(* Logix 5000 Program export IO_Mapping; software revision 30.00; part 2 of 3 *)
(* tags used below, declared in another part *)
   Out_VMAC : DINT[8];
   MajFunc : DINT;
   HashBuffer_H : DINT;
   HashBuffer_G : DINT;
   HashBuffer_F : DINT;
   HashBuffer_E : DINT;
   HashBuffer_D : DINT;
   HashBuffer_C : DINT;
   HashBuffer_B : DINT;
   HashBuffer_A : DINT;
   W : DINT[64];   // MESSAGE SCHEDULE
   tmp : DINT[20];
   T2 : DINT;
   T1 : DINT;
   t : INT;
   M : INT;   // MESSAGE INCREMENTS
   SigmaE : DINT;
   SigmaA : DINT;
   i : INT;
   HashBufferInput_H : DINT;
   HashBufferInput_G : DINT;
   HashBufferInput_F : DINT;
   HashBufferInput_E : DINT;
   HashBufferInput_D : DINT;
   HashBufferInput_C : DINT;
   HashBufferInput_B : DINT;
   HashBufferInput_A : DINT;
   K : DINT[64];
   TOTAL_MSG_LENGTH_MINUS_16 : DINT;
   ROUNDS : DINT;
   n : INT;
(* VMAC, continued *)

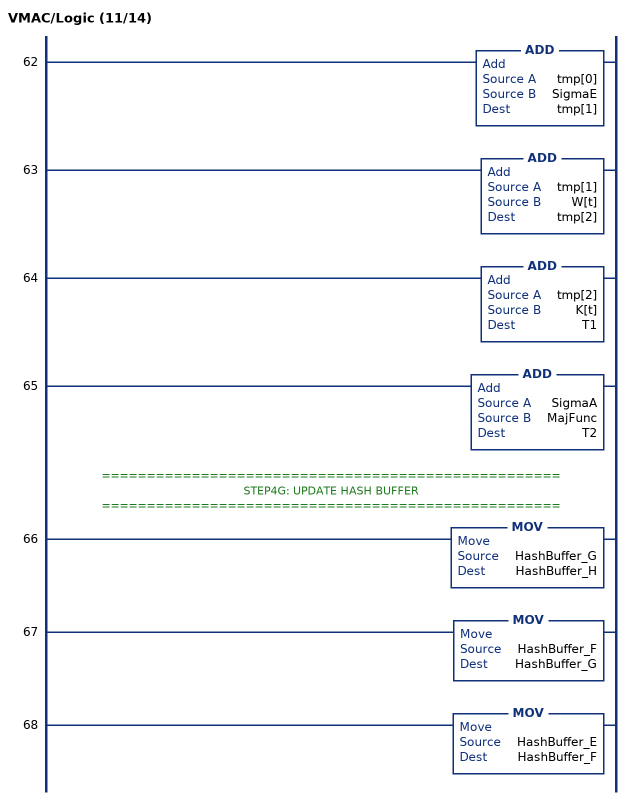
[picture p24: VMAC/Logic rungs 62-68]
   62: ADD(tmp[0],SigmaE,tmp[1]);
   63: ADD(tmp[1],W[t],tmp[2]);
   64: ADD(tmp[2],K[t],T1);
   65: ADD(SigmaA,MajFunc,T2);
   // ===================================================
   // STEP4G: UPDATE HASH BUFFER
   // ===================================================
   66: MOV(HashBuffer_G,HashBuffer_H);
   67: MOV(HashBuffer_F,HashBuffer_G);
   68: MOV(HashBuffer_E,HashBuffer_F);
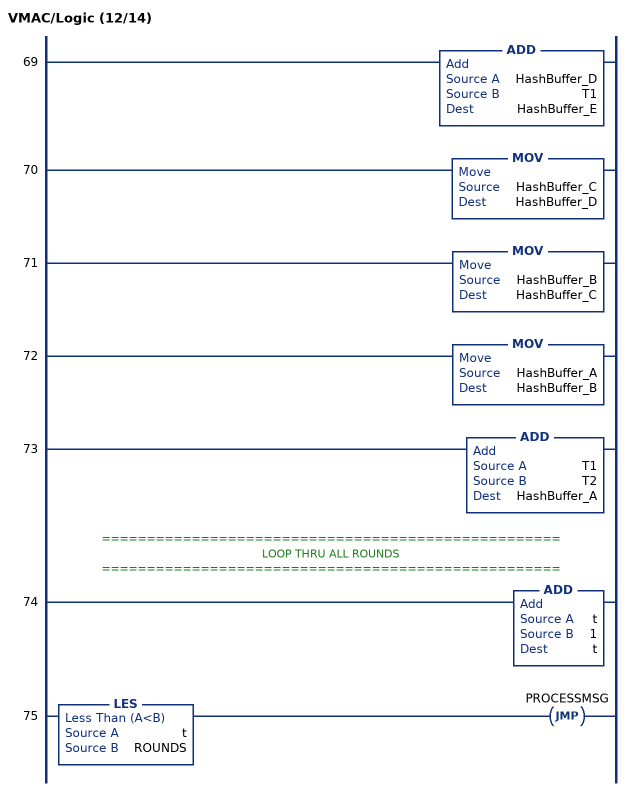
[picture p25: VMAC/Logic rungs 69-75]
   69: ADD(HashBuffer_D,T1,HashBuffer_E);
   70: MOV(HashBuffer_C,HashBuffer_D);
   71: MOV(HashBuffer_B,HashBuffer_C);
   72: MOV(HashBuffer_A,HashBuffer_B);
   73: ADD(T1,T2,HashBuffer_A);
   // ===================================================
   // LOOP THRU ALL ROUNDS
   // ===================================================
   74: ADD(t,1,t);
   75: LES(t,ROUNDS)JMP(PROCESSMSG);
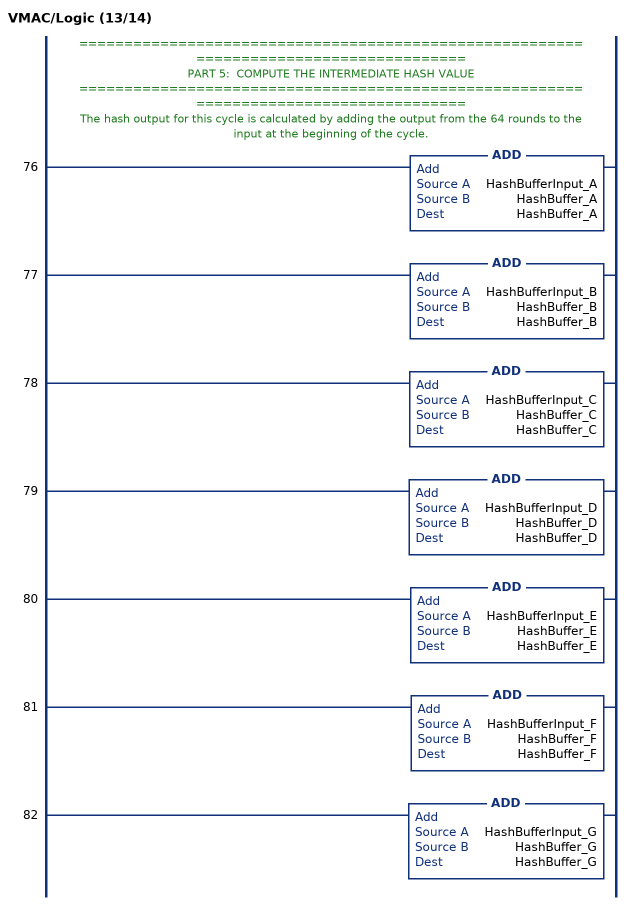
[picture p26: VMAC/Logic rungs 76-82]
   // ======================================================================================
   // PART 5:  COMPUTE THE INTERMEDIATE HASH VALUE
   // ======================================================================================
   // The hash output for this cycle is calculated by adding the output from the 64 rounds to the input at the beginning of the cycle.
   76: ADD(HashBufferInput_A,HashBuffer_A,HashBuffer_A);
   77: ADD(HashBufferInput_B,HashBuffer_B,HashBuffer_B);
   78: ADD(HashBufferInput_C,HashBuffer_C,HashBuffer_C);
   79: ADD(HashBufferInput_D,HashBuffer_D,HashBuffer_D);
   80: ADD(HashBufferInput_E,HashBuffer_E,HashBuffer_E);
   81: ADD(HashBufferInput_F,HashBuffer_F,HashBuffer_F);
   82: ADD(HashBufferInput_G,HashBuffer_G,HashBuffer_G);
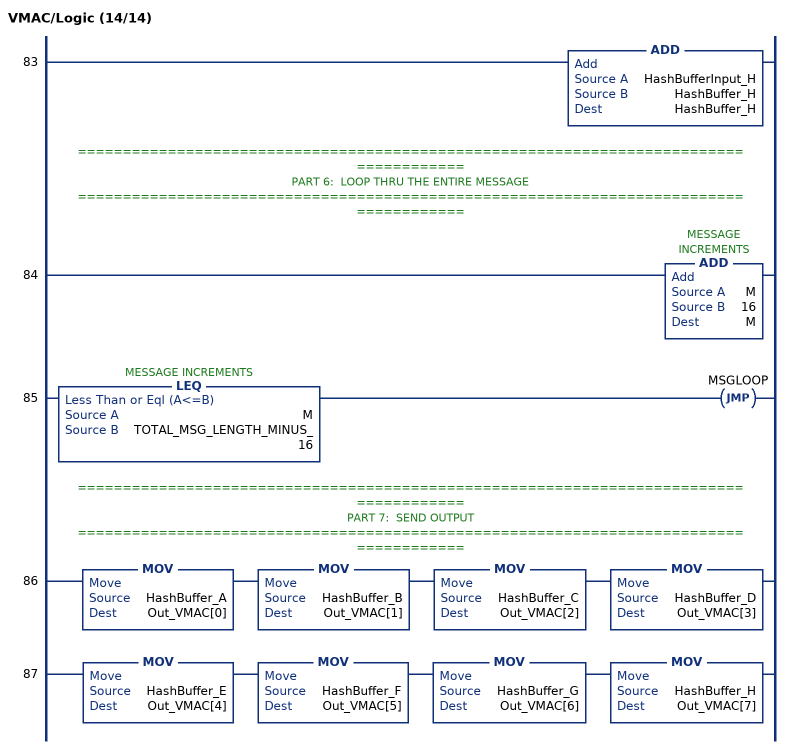
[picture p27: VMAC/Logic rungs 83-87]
   83: ADD(HashBufferInput_H,HashBuffer_H,HashBuffer_H);
   // ======================================================================================
   // PART 6:  LOOP THRU THE ENTIRE MESSAGE
   // ======================================================================================
   84: ADD(M,16,M);
   85: LEQ(M,TOTAL_MSG_LENGTH_MINUS_16)JMP(MSGLOOP);
   // ======================================================================================
   // PART 7:  SEND OUTPUT
   // ======================================================================================
   86: MOV(HashBuffer_A,Out_VMAC[0])MOV(HashBuffer_B,Out_VMAC[1])MOV(HashBuffer_C,Out_VMAC[2])MOV(HashBuffer_D,Out_VMAC[3]);
   87: MOV(HashBuffer_E,Out_VMAC[4])MOV(HashBuffer_F,Out_VMAC[5])MOV(HashBuffer_G,Out_VMAC[6])MOV(HashBuffer_H,Out_VMAC[7]);
END_ROUTINE
END_ADD_ON_INSTRUCTION

ADD_ON_INSTRUCTION L_EQU   (* revision 1.0 01 Release, vendor Rockwell Automation, ExecuteEnableInFalse *)
// Equal (64-bit)
// Revision note:
// Deleted unused Local Tag
// Help:
// This instruction compares two LINT (64-bit signed integer) variables.
// If Inp_A is equal to Inp_B, EnableOut and Out are set to true (1).
// Otherwise EnableOut and Out are cleared to false (0).
VAR_IN_OUT
   Inp_A : LINT; {required}   // Input A
   Inp_B : LINT; {required}   // Input B
END_VAR
VAR_OUTPUT
   Out : BOOL; {access Read Only, visible}   // TRUE if Inp_A is greater than or equal to Inp_B
END_VAR
VAR
   Wrk_Inp_B : DINT[2];   // 32-bit portions of Input B
   Wrk_Inp_A : DINT[2];   // 32-bit portions of Input A
END_VAR

ROUTINE EnableInFalse   (* ladder *)
// If rung is false, clear output "Out"
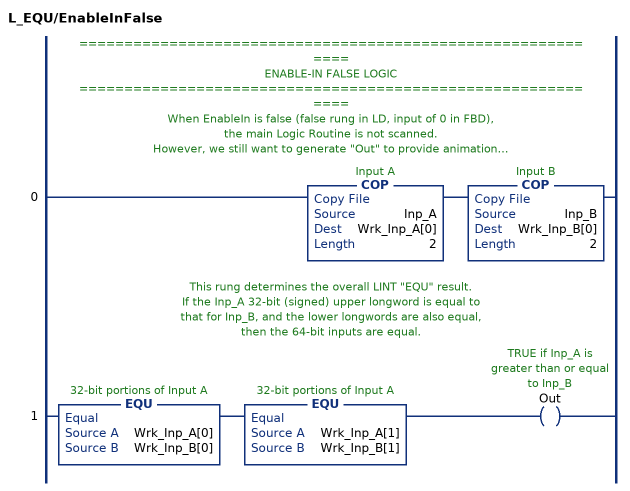
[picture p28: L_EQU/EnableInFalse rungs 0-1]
   // ============================================================
   // ENABLE-IN FALSE LOGIC
   // ============================================================
   // When EnableIn is false (false rung in LD, input of 0 in FBD),
   // the main Logic Routine is not scanned.
   // However, we still want to generate "Out" to provide animation!
   // ===================================================
   // CONVERT LINTs TO DINTs
   // ===================================================
   // These COPies take the input LINTs and break them into a
   // pair of DINTs each.  If the corresponding DINTs (high-order and high-order,
   // and low-order and low-order) are equal, then the input LINTs are equal.
   0: COP(Inp_A,Wrk_Inp_A[0],2)COP(Inp_B,Wrk_Inp_B[0],2);
   // This rung determines the overall LINT "EQU" result.
   // If the Inp_A 32-bit (signed) upper longword is equal to
   // that for Inp_B, and the lower longwords are also equal,
   // then the 64-bit inputs are equal.
   1: EQU(Wrk_Inp_A[0],Wrk_Inp_B[0])EQU(Wrk_Inp_A[1],Wrk_Inp_B[1])OTE(Out);
END_ROUTINE

ROUTINE Logic   (* ladder *)
// Compare inputs and output TRUE if they are equal
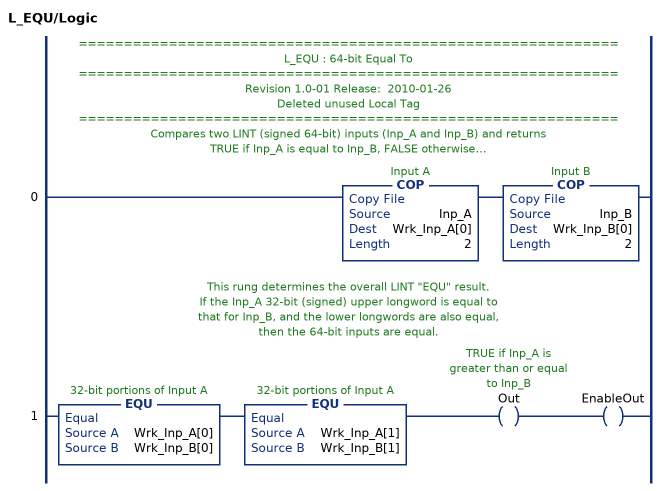
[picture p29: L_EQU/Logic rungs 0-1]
   // ============================================================
   // L_EQU : 64-bit Equal To
   // ============================================================
   // Revision 1.0-01 Release:  2010-01-26
   // Deleted unused Local Tag
   // ============================================================
   // Compares two LINT (signed 64-bit) inputs (Inp_A and Inp_B) and returns
   // TRUE if Inp_A is equal to Inp_B, FALSE otherwise.
   // This instruction breaks each LINT inputs into two DINTs
   // (32 bit signed each) to do the comparison.
   // ===================================================
   // CONVERT LINTs TO DINTs
   // ===================================================
   // These COPies take the input LINTs and break them into a
   // pair of DINTs each.  If the corresponding DINTs (high-order and high-order,
   // and low-order and low-order) are equal, then the input LINTs are equal.
   0: COP(Inp_A,Wrk_Inp_A[0],2)COP(Inp_B,Wrk_Inp_B[0],2);
   // This rung determines the overall LINT "EQU" result.
   // If the Inp_A 32-bit (signed) upper longword is equal to
   // that for Inp_B, and the lower longwords are also equal,
   // then the 64-bit inputs are equal.
   1: EQU(Wrk_Inp_A[0],Wrk_Inp_B[0])EQU(Wrk_Inp_A[1],Wrk_Inp_B[1])OTE(Out)OTE(EnableOut);
END_ROUTINE
END_ADD_ON_INSTRUCTION

ADD_ON_INSTRUCTION L_LES   (* revision 1.1 20170624, vendor Ken Fischer, NSWCPD, C516, ExecuteEnableInFalse *)
// Less Than (64-bit)
// Revision note:
// Rev1.1:  20170624 - Corrected comment on the Out bit
// Help:
// This instruction compares two LINT (64-bit signed integer) variables.
// If Inp_A is less than Inp_B, EnableOut and Out are set to true (1).
// Otherwise EnableOut and Out are cleared to false (0).
VAR_IN_OUT
   Inp_A : LINT; {required}   // Input A
   Inp_B : LINT; {required}   // Input B
END_VAR
VAR_OUTPUT
   Out : BOOL; {access Read Only, visible}   // TRUE if Inp_A is less than Inp_B
END_VAR
VAR
   Wrk_Inp_B : DINT[4];   // 32-bit portions of Input B
   Wrk_Inp_A : DINT[4];   // 32-bit portions of Input A
END_VAR

ROUTINE EnableInFalse   (* ladder *)
// If rung is false, clear output "Out"
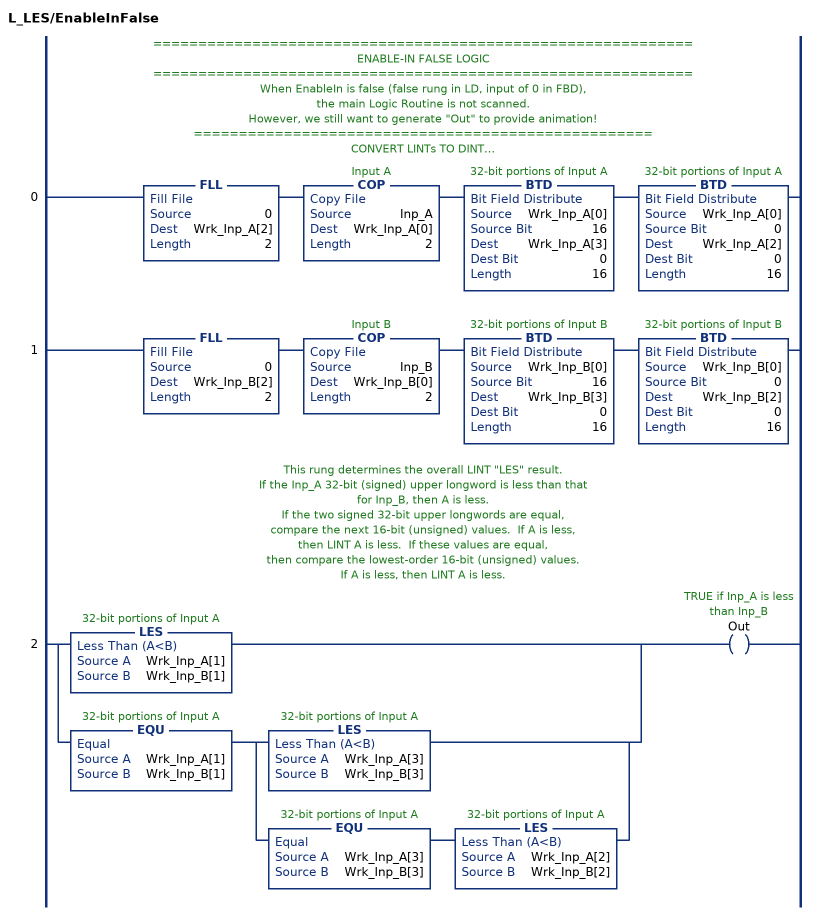
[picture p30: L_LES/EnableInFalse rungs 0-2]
   // ============================================================
   // ENABLE-IN FALSE LOGIC
   // ============================================================
   // When EnableIn is false (false rung in LD, input of 0 in FBD),
   // the main Logic Routine is not scanned.
   // However, we still want to generate "Out" to provide animation!
   // ===================================================
   // CONVERT LINTs TO DINTs
   // ===================================================
   // These COPies and BTDs take the input LINTs and break them into a
   // pair of DINTs each, then take the low-order signed DINT and breaks it
   // further into two 16-bit values so we can do unsigned compares on them.
   // Logix V17 has a LINT data type, but math instructions
   // (and AOI Input and Output Parameters) don't support LINT.
   0: FLL(0,Wrk_Inp_A[2],2)COP(Inp_A,Wrk_Inp_A[0],2)BTD(Wrk_Inp_A[0],16,Wrk_Inp_A[3],0,16)BTD(Wrk_Inp_A[0],0,Wrk_Inp_A[2],0,16);
   1: FLL(0,Wrk_Inp_B[2],2)COP(Inp_B,Wrk_Inp_B[0],2)BTD(Wrk_Inp_B[0],16,Wrk_Inp_B[3],0,16)BTD(Wrk_Inp_B[0],0,Wrk_Inp_B[2],0,16);
   // This rung determines the overall LINT "LES" result.
   // If the Inp_A 32-bit (signed) upper longword is less than that
   // for Inp_B, then A is less.
   // If the two signed 32-bit upper longwords are equal,
   // compare the next 16-bit (unsigned) values.  If A is less,
   // then LINT A is less.  If these values are equal,
   // then compare the lowest-order 16-bit (unsigned) values.
   // If A is less, then LINT A is less.
   2: [LES(Wrk_Inp_A[1],Wrk_Inp_B[1]) ,EQU(Wrk_Inp_A[1],Wrk_Inp_B[1]) [LES(Wrk_Inp_A[3],Wrk_Inp_B[3]) ,EQU(Wrk_Inp_A[3],Wrk_Inp_B[3]) LES(Wrk_Inp_A[2],Wrk_Inp_B[2]) ] ]OTE(Out);
END_ROUTINE

ROUTINE Logic   (* ladder *)
// Compare inputs and output TRUE if Inp_A < Inp_B
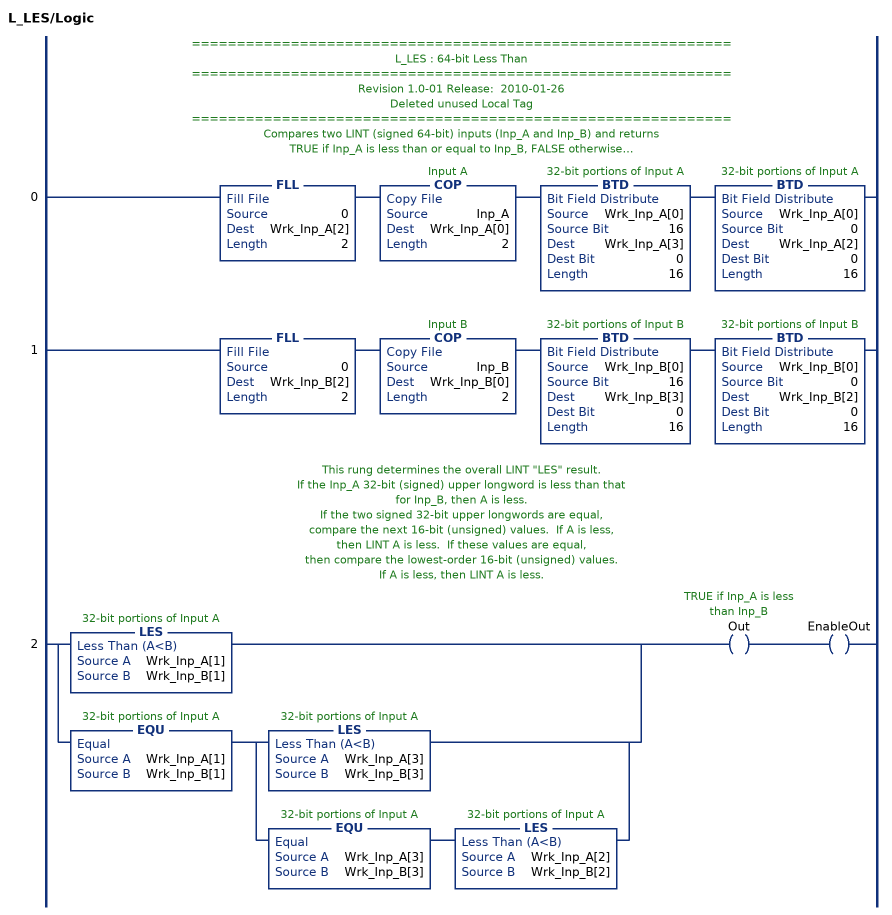
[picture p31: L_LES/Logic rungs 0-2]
   // ============================================================
   // L_LES : 64-bit Less Than
   // ============================================================
   // Revision 1.0-01 Release:  2010-01-26
   // Deleted unused Local Tag
   // ============================================================
   // Compares two LINT (signed 64-bit) inputs (Inp_A and Inp_B) and returns
   // TRUE if Inp_A is less than or equal to Inp_B, FALSE otherwise.
   // This instruction breaks the LINT inputs into three DINTs
   // (32 bit signed, 16 bit unsigned and 16 bit unsigned) to do the comparison.
   // ===================================================
   // CONVERT LINTs TO DINTs
   // ===================================================
   // These COPies and BTDs take the input LINTs and break them into a
   // pair of DINTs each, then take the low-order signed DINT and breaks it
   // further into two 16-bit values so we can do unsigned compares on them.
   // Logix V17 has a LINT data type, but math instructions
   // (and AOI Input and Output Parameters) don't support LINT.
   0: FLL(0,Wrk_Inp_A[2],2)COP(Inp_A,Wrk_Inp_A[0],2)BTD(Wrk_Inp_A[0],16,Wrk_Inp_A[3],0,16)BTD(Wrk_Inp_A[0],0,Wrk_Inp_A[2],0,16);
   1: FLL(0,Wrk_Inp_B[2],2)COP(Inp_B,Wrk_Inp_B[0],2)BTD(Wrk_Inp_B[0],16,Wrk_Inp_B[3],0,16)BTD(Wrk_Inp_B[0],0,Wrk_Inp_B[2],0,16);
   // This rung determines the overall LINT "LES" result.
   // If the Inp_A 32-bit (signed) upper longword is less than that
   // for Inp_B, then A is less.
   // If the two signed 32-bit upper longwords are equal,
   // compare the next 16-bit (unsigned) values.  If A is less,
   // then LINT A is less.  If these values are equal,
   // then compare the lowest-order 16-bit (unsigned) values.
   // If A is less, then LINT A is less.
   2: [LES(Wrk_Inp_A[1],Wrk_Inp_B[1]) ,EQU(Wrk_Inp_A[1],Wrk_Inp_B[1]) [LES(Wrk_Inp_A[3],Wrk_Inp_B[3]) ,EQU(Wrk_Inp_A[3],Wrk_Inp_B[3]) LES(Wrk_Inp_A[2],Wrk_Inp_B[2]) ] ]OTE(Out)OTE(EnableOut);
END_ROUTINE
END_ADD_ON_INSTRUCTION

ADD_ON_INSTRUCTION L_MOV   (* revision 1.0 20170709, vendor Ken Fischer, NSWCPD, C516 *)
// MOV (64-bit)
// Revision note:
// Initial Release
// Help:
// Adds two LINT (signed 64-bit) values and returns a LINT (signed 64-bit) sum.
// Also provides math status bits for Carry, Negative, Overflow and Zero result
// (equivalent to built-in S:C, S:N, S:V, S:Z).
VAR_IN_OUT
   Inp : LINT; {required}   // First Addend, 64-bit Integer
   Out : LINT; {required}   // Sum, 64-bit Integer
END_VAR
VAR
   Wrk : DINT[2];   // Input A as two 32-bit DINTs
END_VAR

ROUTINE Logic   (* ladder *)
// Do 64-bit addition
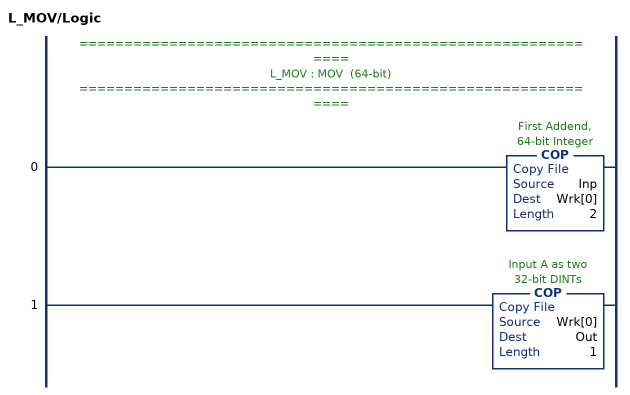
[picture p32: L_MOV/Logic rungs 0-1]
   // ============================================================
   // L_MOV : MOV  (64-bit)
   // ============================================================
   0: COP(Inp,Wrk[0],2);
   1: COP(Wrk[0],Out,1);
END_ROUTINE
END_ADD_ON_INSTRUCTION

VAR_GLOBAL   (* controller tags *)
   DATA_MSG_NODE1 : VMAC_DATA_MSG := (STATUS.RunMode := 1, DATA[0] := -1255628806, DATA[1] := 205831, DATA[2] := 1, DATA[3] := 234, LEN := 100, ROUNDS := 20, VMAC[0] := 16#7492_4488, VMAC[1] := 16#f3d9_1e52, VMAC[2] := 16#4fd4_cec1, VMAC[3] := 16#69d5_423d, VMAC[4] := 16#3008_6ba3, VMAC[5] := 16#7997_d6e6, VMAC[6] := 16#041b_b1f3, VMAC[7] := 16#c3f5_4f2d); {produced}
        ProduceInfo(ProduceCount := 10)
   DATA_MSG_NODE2 : VMAC_DATA_MSG := (STATUS.RunMode := 1, DATA[0] := -417090202, DATA[1] := 205750, DATA[2] := 2, DATA[3] := 134, DATA[54] := -2147483648, DATA[63] := 1728, LEN := 100, ROUNDS := 20, VMAC[0] := 16#24c4_fa25, VMAC[1] := 16#6eff_3326, VMAC[2] := 16#3282_7ac5, VMAC[3] := 16#2ca0_e4c9, VMAC[4] := 16#bf5d_a1c2, VMAC[5] := 16#4aa7_7c3d, VMAC[6] := 16#31bc_bb48, VMAC[7] := 16#60fa_c975); {consumed}
        ConsumeInfo(Producer := NODE2, RemoteTag := DATA_MSG_NODE2, RemoteInstance := 0, RPI := 20)
   DATA_MSG_NODE3 : VMAC_DATA_MSG := (STATUS.RunMode := 1, DATA[0] := -4597227, DATA[1] := 205750, DATA[2] := 3, DATA[3] := 124, DATA[26] := -2147483648, DATA[31] := 832, LEN := 100, ROUNDS := 20, VMAC[0] := 16#ed9d_2f40, VMAC[1] := 16#89af_0d05, VMAC[2] := 16#f8ea_c0f1, VMAC[3] := 16#9e30_7597, VMAC[4] := 16#0f86_4794, VMAC[5] := 16#f7e1_da30, VMAC[6] := 16#df2a_caef, VMAC[7] := 16#b2ab_3103); {consumed}
        ConsumeInfo(Producer := NODE3, RemoteTag := DATA_MSG_NODE3, RemoteInstance := 0, RPI := 20)
   DATA_MSG_NODE4 : VMAC_DATA_MSG := (STATUS.RunMode := 1, DATA[0] := 476192980, DATA[1] := 205751, DATA[2] := 4, DATA[3] := 123, DATA[40] := -2147483648, DATA[47] := 1280, LEN := 100, ROUNDS := 20, VMAC[0] := 16#f777_7f49, VMAC[1] := 16#51db_2182, VMAC[2] := 16#8ec3_09ae, VMAC[3] := 16#8a45_334b, VMAC[4] := 16#e7f0_7395, VMAC[5] := 16#2d59_0226, VMAC[6] := 16#4e52_3ff8, VMAC[7] := 16#02fe_9964); {consumed}
        ConsumeInfo(Producer := NODE4, RemoteTag := DATA_MSG_NODE4, RemoteInstance := 0, RPI := 20)
   EdDSA_KS : DINT[8];
   EdDSA_KS_Prime : DINT[8];
   InternalFlag_AllNodesHaveMyKsPrime : BOOL;
   InternalFlag_KsID : LINT;
   InternalFlag_KsPrimeID : LINT;
   KAF_COMMS_UP : BOOL := 1;   // TEMP TAG
   NODE : VMAC_DATA_INTERNAL[5];
   VMAC_KEY : DINT[8] := ([0] := -14421854, [1] := 1732551659, [2] := 1179356203, [3] := -1910315757, [4] := -1017021417, [5] := 1555248667, [6] := 1414909173, [7] := 1770998633);
   VMAC_KEY_ID : LINT;
   Wrk_InpA : DINT[2];
   Wrk_InpB : DINT[2];
END_VAR

PROGRAM IO_Mapping   (* main routine MainRoutine *)
VAR
   B256_CtoE : B256_CtoE;
   B256_EtoDINT : B256_EtoDINT;
   B256_StoC : B256_StoC;
   ledtemp : INT;
   L_INC : L_INC;
   L_MOV : L_MOV;
   TEMP : INT := 16384;
   Temp_C : DINT[22];
   Temp_E : DINT[32];
END_VAR

ROUTINE AI_Mapping   (* ladder *)
   0: NOP();
END_ROUTINE

ROUTINE AO_Mapping   (* ladder *)
   0: NOP();
END_ROUTINE

ROUTINE DI_Mapping   (* ladder *)
   0: NOP();
END_ROUTINE

ROUTINE DO_Mapping   (* ladder *)
   0: NOP();
END_ROUTINE

ROUTINE MainRoutine   (* ladder *)
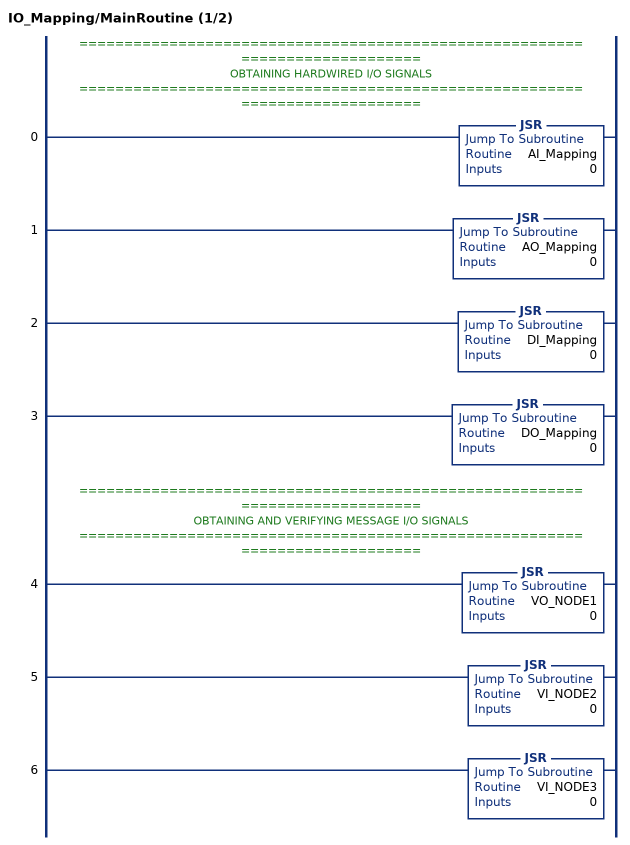
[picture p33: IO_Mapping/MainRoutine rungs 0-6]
   // ============================================================================
   // OBTAINING HARDWIRED I/O SIGNALS
   // ============================================================================
   0: JSR(AI_Mapping,0);
   1: JSR(AO_Mapping,0);
   2: JSR(DI_Mapping,0);
   3: JSR(DO_Mapping,0);
   // ============================================================================
   // OBTAINING AND VERIFYING MESSAGE I/O SIGNALS
   // ============================================================================
   4: JSR(VO_NODE1,0);
   5: JSR(VI_NODE2,0);
   6: JSR(VI_NODE3,0);
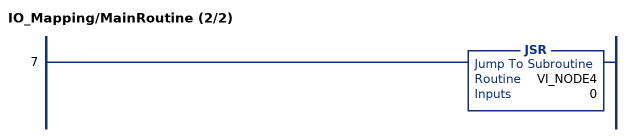
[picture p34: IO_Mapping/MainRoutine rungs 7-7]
   7: JSR(VI_NODE4,0);
END_ROUTINE

ROUTINE VI_NODE2   (* ladder *)
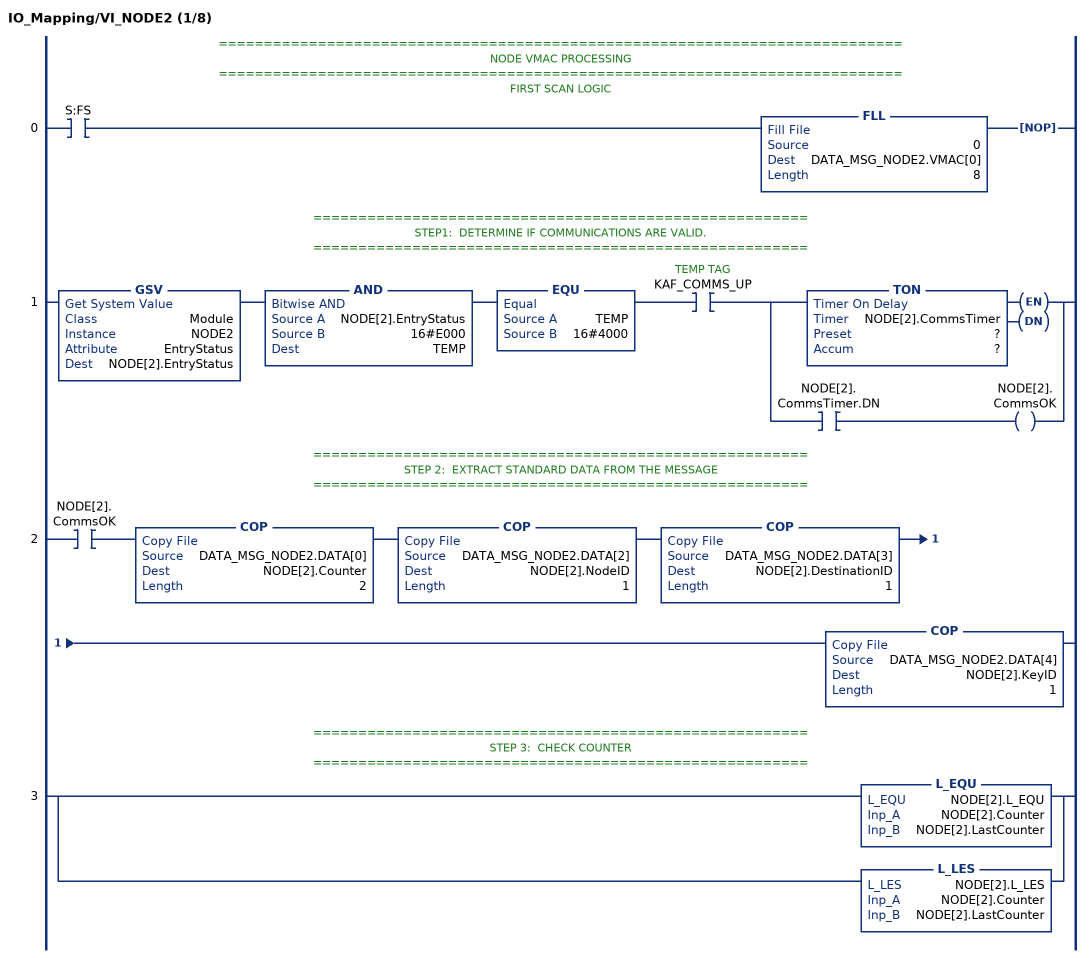
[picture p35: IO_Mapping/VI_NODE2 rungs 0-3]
   // ============================================================================
   // NODE VMAC PROCESSING
   // ============================================================================
   // FIRST SCAN LOGIC
   0: XIC(S:FS)FLL(0,DATA_MSG_NODE2.VMAC[0],8)NOP();
   // =======================================================
   // STEP1:  DETERMINE IF COMMUNICATIONS ARE VALID.
   // =======================================================
   1: GSV(Module,NODE2,EntryStatus,NODE[2].EntryStatus)AND(NODE[2].EntryStatus,16#E000,TEMP)EQU(TEMP,16#4000)XIC(KAF_COMMS_UP)[TON(NODE[2].CommsTimer,?,?) ,XIC(NODE[2].CommsTimer.DN) OTE(NODE[2].CommsOK) ];
   // =======================================================
   // STEP 2:  EXTRACT STANDARD DATA FROM THE MESSAGE
   // =======================================================
   2: XIC(NODE[2].CommsOK)COP(DATA_MSG_NODE2.DATA[0],NODE[2].Counter,2)COP(DATA_MSG_NODE2.DATA[2],NODE[2].NodeID,1)COP(DATA_MSG_NODE2.DATA[3],NODE[2].DestinationID,1)COP(DATA_MSG_NODE2.DATA[4],NODE[2].KeyID,1);
   // =======================================================
   // STEP 3:  CHECK COUNTER
   // =======================================================
   3: [L_EQU(NODE[2].L_EQU,NODE[2].Counter,NODE[2].LastCounter) ,L_LES(NODE[2].L_LES,NODE[2].Counter,NODE[2].LastCounter) ];
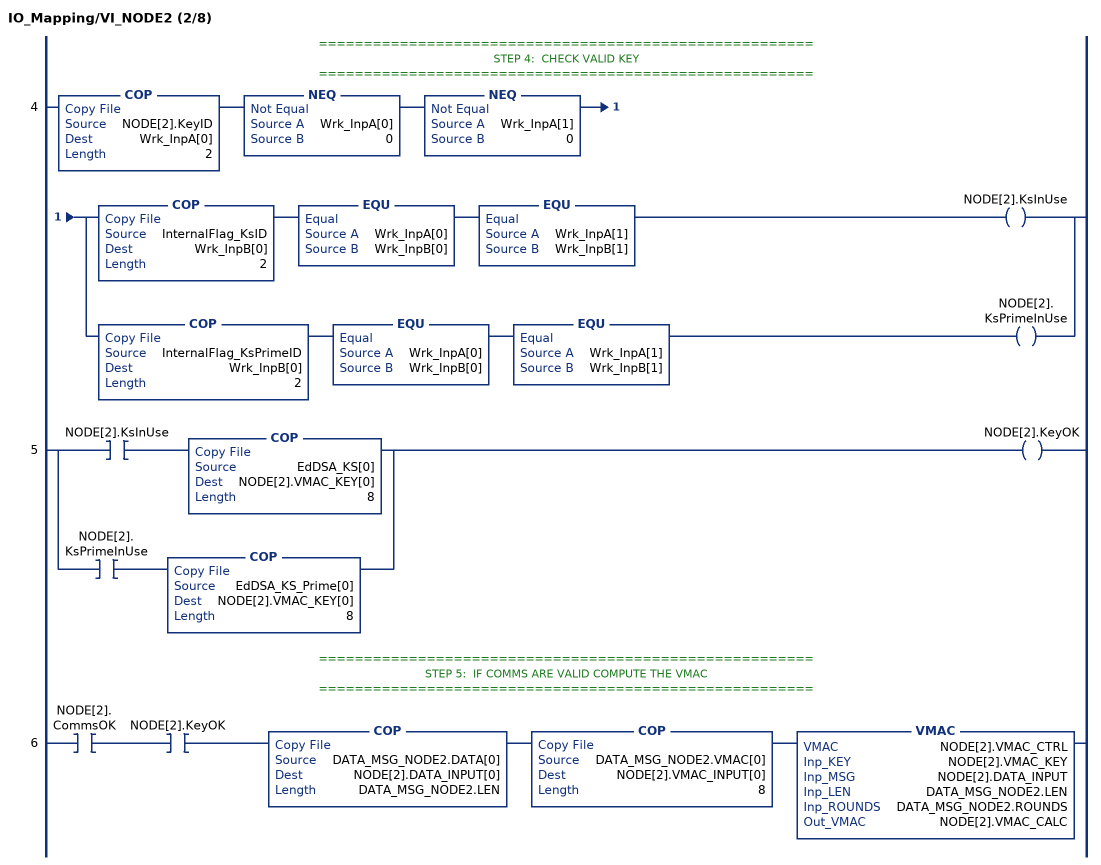
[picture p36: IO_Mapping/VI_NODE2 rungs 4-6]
   // =======================================================
   // STEP 4:  CHECK VALID KEY
   // =======================================================
   4: COP(NODE[2].KeyID,Wrk_InpA[0],2)NEQ(Wrk_InpA[0],0)NEQ(Wrk_InpA[1],0)[COP(InternalFlag_KsID,Wrk_InpB[0],2) EQU(Wrk_InpA[0],Wrk_InpB[0]) EQU(Wrk_InpA[1],Wrk_InpB[1]) OTE(NODE[2].KsInUse) ,COP(InternalFlag_KsPrimeID,Wrk_InpB[0],2) EQU(Wrk_InpA[0],Wrk_InpB[0]) EQU(Wrk_InpA[1],Wrk_InpB[1]) OTE(NODE[2].KsPrimeInUse) ];
   5: [XIC(NODE[2].KsInUse) COP(EdDSA_KS[0],NODE[2].VMAC_KEY[0],8) ,XIC(NODE[2].KsPrimeInUse) COP(EdDSA_KS_Prime[0],NODE[2].VMAC_KEY[0],8) ]OTE(NODE[2].KeyOK);
   // =======================================================
   // STEP 5:  IF COMMS ARE VALID COMPUTE THE VMAC
   // =======================================================
   6: XIC(NODE[2].CommsOK)XIC(NODE[2].KeyOK)COP(DATA_MSG_NODE2.DATA[0],NODE[2].DATA_INPUT[0],DATA_MSG_NODE2.LEN)COP(DATA_MSG_NODE2.VMAC[0],NODE[2].VMAC_INPUT[0],8)VMAC(NODE[2].VMAC_CTRL,NODE[2].VMAC_KEY,NODE[2].DATA_INPUT,DATA_MSG_NODE2.LEN,DATA_MSG_NODE2.ROUNDS,NODE[2].VMAC_CALC);
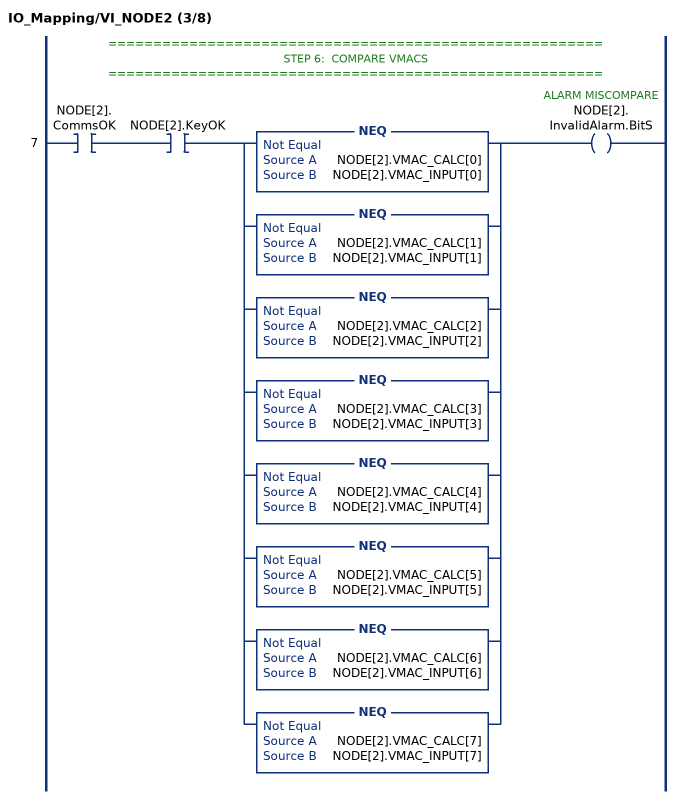
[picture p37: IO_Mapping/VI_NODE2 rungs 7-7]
   // =======================================================
   // STEP 6:  COMPARE VMACS
   // =======================================================
   7: XIC(NODE[2].CommsOK)XIC(NODE[2].KeyOK)[NEQ(NODE[2].VMAC_CALC[0],NODE[2].VMAC_INPUT[0]) ,NEQ(NODE[2].VMAC_CALC[1],NODE[2].VMAC_INPUT[1]) ,NEQ(NODE[2].VMAC_CALC[2],NODE[2].VMAC_INPUT[2]) ,NEQ(NODE[2].VMAC_CALC[3],NODE[2].VMAC_INPUT[3]) ,NEQ(NODE[2].VMAC_CALC[4],NODE[2].VMAC_INPUT[4]) ,NEQ(NODE[2].VMAC_CALC[5],NODE[2].VMAC_INPUT[5]) ,NEQ(NODE[2].VMAC_CALC[6],NODE[2].VMAC_INPUT[6]) ,NEQ(NODE[2].VMAC_CALC[7],NODE[2].VMAC_INPUT[7]) ]OTE(NODE[2].InvalidAlarm.BitS);
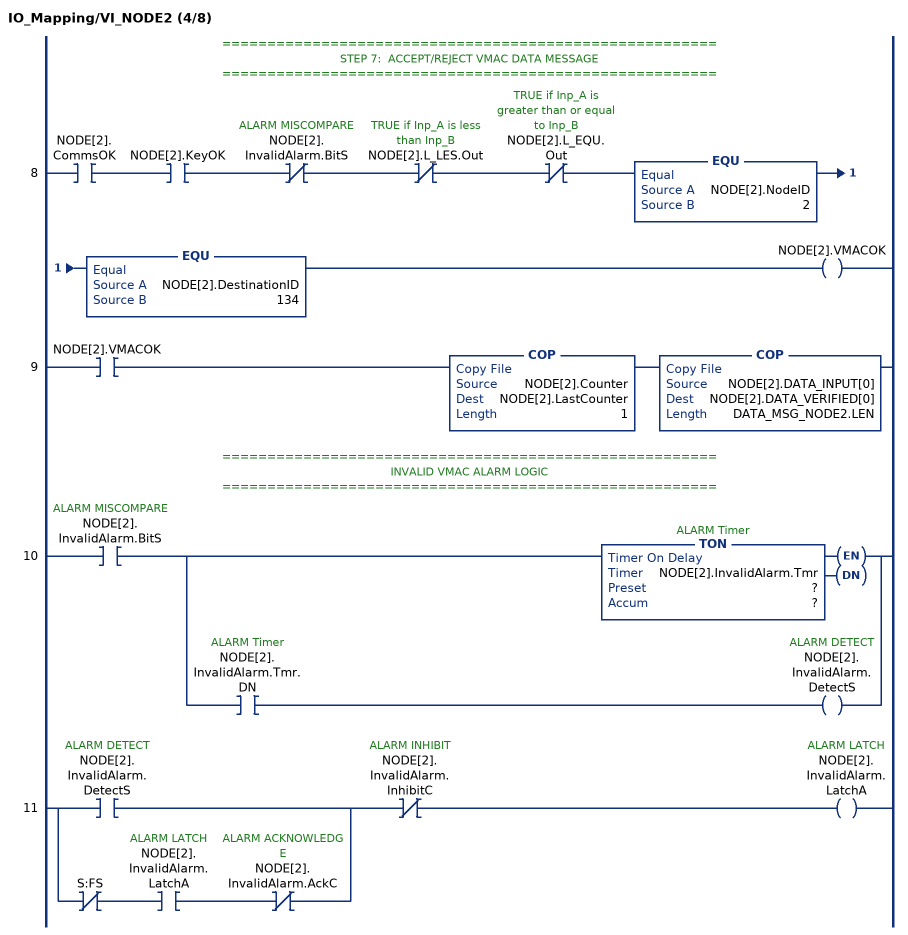
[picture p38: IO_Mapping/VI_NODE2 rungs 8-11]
   // =======================================================
   // STEP 7:  ACCEPT/REJECT VMAC DATA MESSAGE
   // =======================================================
   8: XIC(NODE[2].CommsOK)XIC(NODE[2].KeyOK)XIO(NODE[2].InvalidAlarm.BitS)XIO(NODE[2].L_LES.Out)XIO(NODE[2].L_EQU.Out)EQU(NODE[2].NodeID,2)EQU(NODE[2].DestinationID,134)OTE(NODE[2].VMACOK);
   9: XIC(NODE[2].VMACOK)COP(NODE[2].Counter,NODE[2].LastCounter,1)COP(NODE[2].DATA_INPUT[0],NODE[2].DATA_VERIFIED[0],DATA_MSG_NODE2.LEN);
   // =======================================================
   // INVALID VMAC ALARM LOGIC
   // =======================================================
   10: XIC(NODE[2].InvalidAlarm.BitS)[TON(NODE[2].InvalidAlarm.Tmr,?,?) ,XIC(NODE[2].InvalidAlarm.Tmr.DN) OTE(NODE[2].InvalidAlarm.DetectS) ];
   11: [XIC(NODE[2].InvalidAlarm.DetectS) ,XIO(S:FS) XIC(NODE[2].InvalidAlarm.LatchA) XIO(NODE[2].InvalidAlarm.AckC) ]XIO(NODE[2].InvalidAlarm.InhibitC)OTE(NODE[2].InvalidAlarm.LatchA);
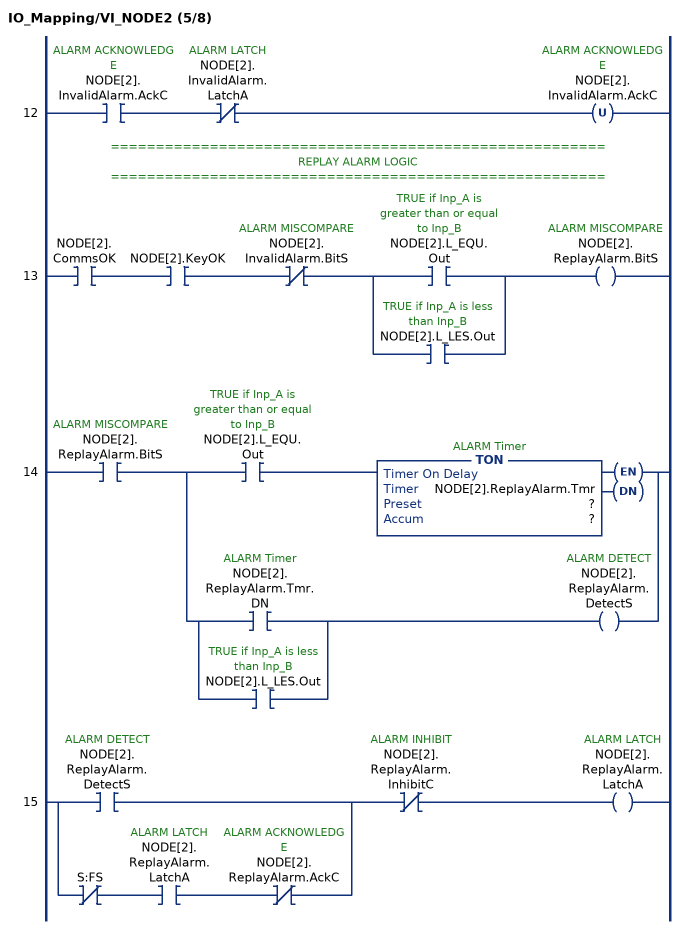
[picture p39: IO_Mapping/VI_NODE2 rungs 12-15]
   12: XIC(NODE[2].InvalidAlarm.AckC)XIO(NODE[2].InvalidAlarm.LatchA)OTU(NODE[2].InvalidAlarm.AckC);
   // =======================================================
   // REPLAY ALARM LOGIC
   // =======================================================
   13: XIC(NODE[2].CommsOK)XIC(NODE[2].KeyOK)XIO(NODE[2].InvalidAlarm.BitS)[XIC(NODE[2].L_EQU.Out) ,XIC(NODE[2].L_LES.Out) ]OTE(NODE[2].ReplayAlarm.BitS);
   14: XIC(NODE[2].ReplayAlarm.BitS)[XIC(NODE[2].L_EQU.Out) TON(NODE[2].ReplayAlarm.Tmr,?,?) ,[XIC(NODE[2].ReplayAlarm.Tmr.DN) ,XIC(NODE[2].L_LES.Out) ] OTE(NODE[2].ReplayAlarm.DetectS) ];
   15: [XIC(NODE[2].ReplayAlarm.DetectS) ,XIO(S:FS) XIC(NODE[2].ReplayAlarm.LatchA) XIO(NODE[2].ReplayAlarm.AckC) ]XIO(NODE[2].ReplayAlarm.InhibitC)OTE(NODE[2].ReplayAlarm.LatchA);
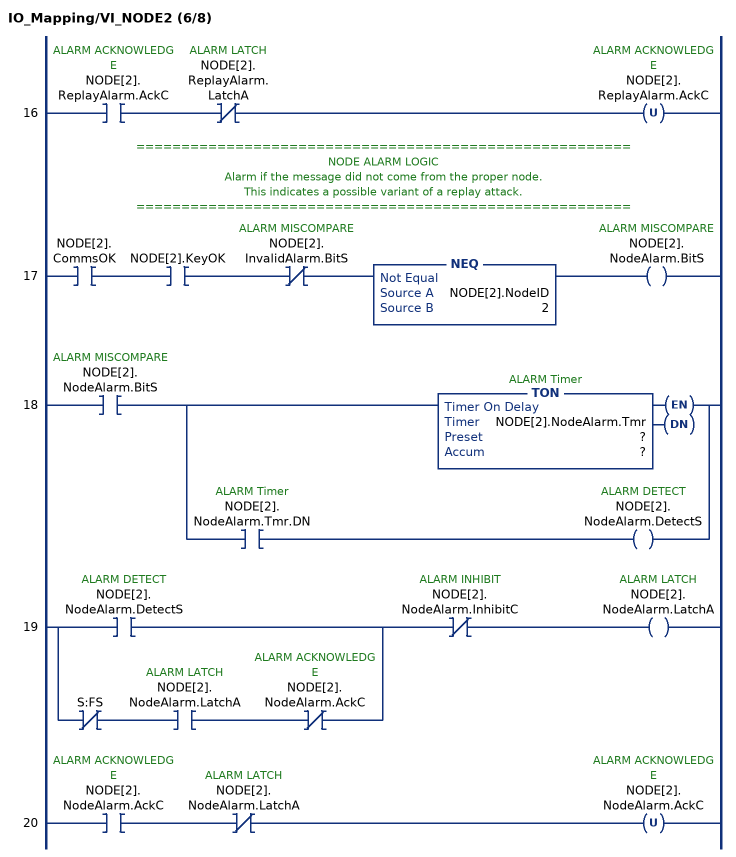
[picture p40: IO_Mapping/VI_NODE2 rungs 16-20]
   16: XIC(NODE[2].ReplayAlarm.AckC)XIO(NODE[2].ReplayAlarm.LatchA)OTU(NODE[2].ReplayAlarm.AckC);
   // =======================================================
   // NODE ALARM LOGIC
   // Alarm if the message did not come from the proper node.
   // This indicates a possible variant of a replay attack.
   // =======================================================
   17: XIC(NODE[2].CommsOK)XIC(NODE[2].KeyOK)XIO(NODE[2].InvalidAlarm.BitS)NEQ(NODE[2].NodeID,2)OTE(NODE[2].NodeAlarm.BitS);
   18: XIC(NODE[2].NodeAlarm.BitS)[TON(NODE[2].NodeAlarm.Tmr,?,?) ,XIC(NODE[2].NodeAlarm.Tmr.DN) OTE(NODE[2].NodeAlarm.DetectS) ];
   19: [XIC(NODE[2].NodeAlarm.DetectS) ,XIO(S:FS) XIC(NODE[2].NodeAlarm.LatchA) XIO(NODE[2].NodeAlarm.AckC) ]XIO(NODE[2].NodeAlarm.InhibitC)OTE(NODE[2].NodeAlarm.LatchA);
   20: XIC(NODE[2].NodeAlarm.AckC)XIO(NODE[2].NodeAlarm.LatchA)OTU(NODE[2].NodeAlarm.AckC);
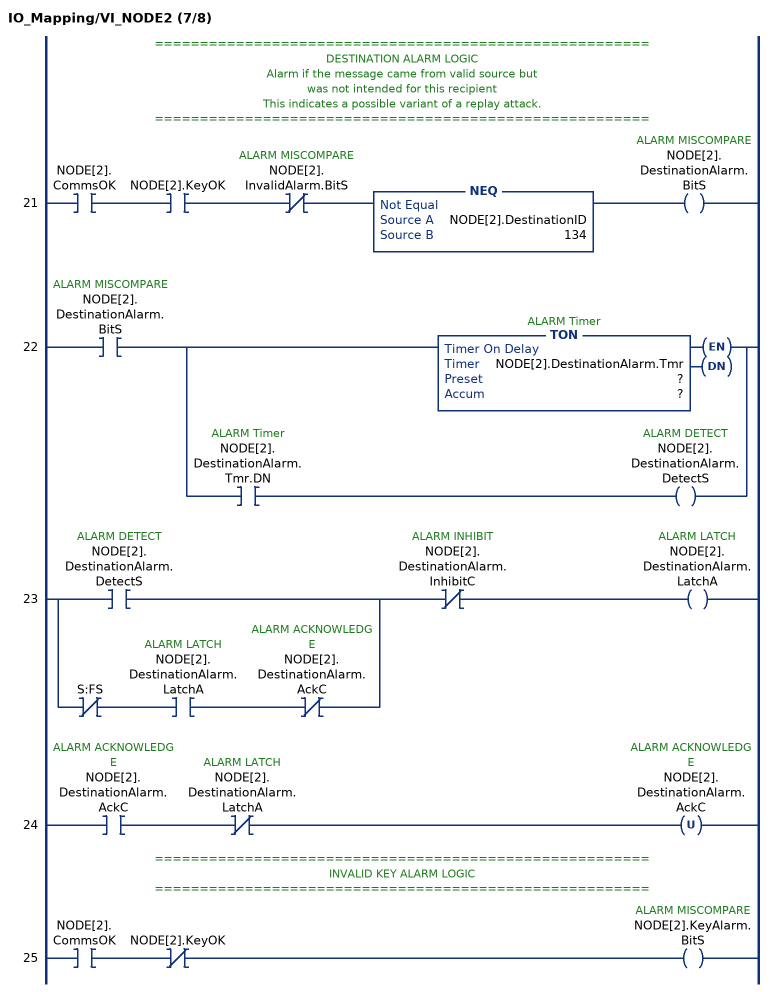
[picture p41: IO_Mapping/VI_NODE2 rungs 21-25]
   // =======================================================
   // DESTINATION ALARM LOGIC
   // Alarm if the message came from valid source but
   // was not intended for this recipient
   // This indicates a possible variant of a replay attack.
   // =======================================================
   21: XIC(NODE[2].CommsOK)XIC(NODE[2].KeyOK)XIO(NODE[2].InvalidAlarm.BitS)NEQ(NODE[2].DestinationID,134)OTE(NODE[2].DestinationAlarm.BitS);
   22: XIC(NODE[2].DestinationAlarm.BitS)[TON(NODE[2].DestinationAlarm.Tmr,?,?) ,XIC(NODE[2].DestinationAlarm.Tmr.DN) OTE(NODE[2].DestinationAlarm.DetectS) ];
   23: [XIC(NODE[2].DestinationAlarm.DetectS) ,XIO(S:FS) XIC(NODE[2].DestinationAlarm.LatchA) XIO(NODE[2].DestinationAlarm.AckC) ]XIO(NODE[2].DestinationAlarm.InhibitC)OTE(NODE[2].DestinationAlarm.LatchA);
   24: XIC(NODE[2].DestinationAlarm.AckC)XIO(NODE[2].DestinationAlarm.LatchA)OTU(NODE[2].DestinationAlarm.AckC);
   // =======================================================
   // INVALID KEY ALARM LOGIC
   // =======================================================
   25: XIC(NODE[2].CommsOK)XIO(NODE[2].KeyOK)OTE(NODE[2].KeyAlarm.BitS);
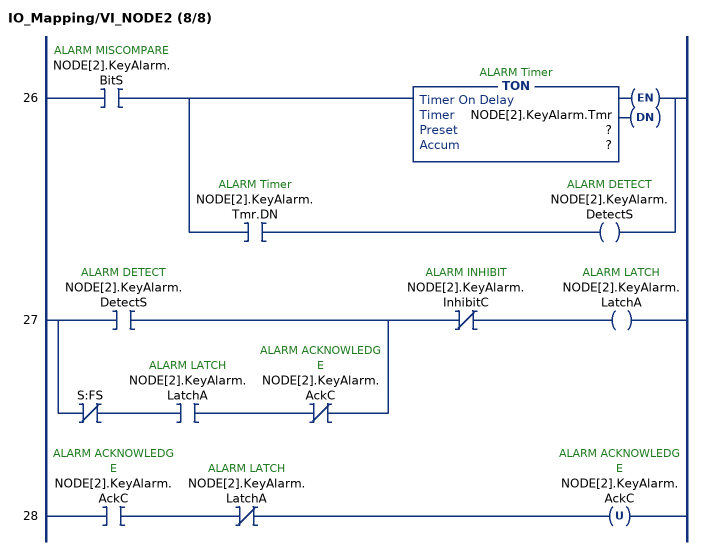
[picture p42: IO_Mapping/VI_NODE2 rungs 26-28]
   26: XIC(NODE[2].KeyAlarm.BitS)[TON(NODE[2].KeyAlarm.Tmr,?,?) ,XIC(NODE[2].KeyAlarm.Tmr.DN) OTE(NODE[2].KeyAlarm.DetectS) ];
   27: [XIC(NODE[2].KeyAlarm.DetectS) ,XIO(S:FS) XIC(NODE[2].KeyAlarm.LatchA) XIO(NODE[2].KeyAlarm.AckC) ]XIO(NODE[2].KeyAlarm.InhibitC)OTE(NODE[2].KeyAlarm.LatchA);
   28: XIC(NODE[2].KeyAlarm.AckC)XIO(NODE[2].KeyAlarm.LatchA)OTU(NODE[2].KeyAlarm.AckC);
END_ROUTINE
